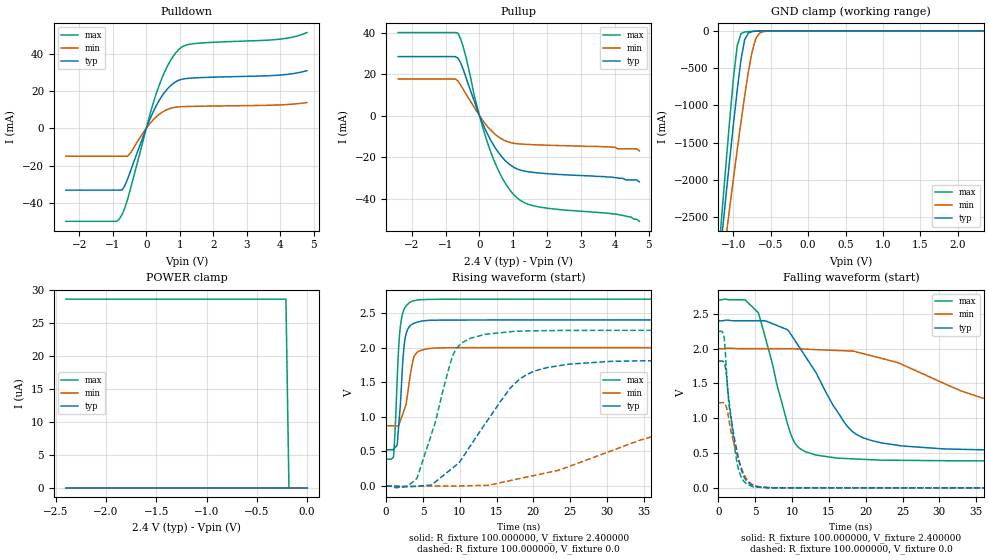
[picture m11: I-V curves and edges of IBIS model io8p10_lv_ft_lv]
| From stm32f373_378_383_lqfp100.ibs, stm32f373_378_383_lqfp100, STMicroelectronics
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|   Model io8p10_lv_ft_lv
[Model]  io8p10_lv_ft_lv
Model_type I/O
Polarity   Non-Inverting
Enable   Active-Low
Vinl =   0.720000V
Vinh =   1.680000V
Vmeas =  1.200000V
Cref =   50.000000pF
Rref =   100.000000M
Vref =   0.0V
C_comp   5.024800pF   4.846300pF   5.260300pF
[Temperature Range]   25.000000   0.125000k   -40.000000
[Pullup Reference]   2.400000V   2.000000V   2.700000V
[Pulldown Reference]   0.0V   0.0V   0.0V
[POWER Clamp Reference]   2.400000V   2.000000V   2.700000V
[GND Clamp Reference]   0.0V   0.0V   0.0V
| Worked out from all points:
|   slope of the pulldown table from 0 to 0.36 V, typ, clamps not added: 25.5 ohm
|   slope of the pullup table from 0 to 0.36 V, typ, clamps not added: 28.4 ohm
|   GND clamp passes 1 mA (typ) near -0.60 V on its own axis
|   rising waveform, R_fixture 100.000000, V_fixture 2.400000: 20-80 % time 716ps typ, 1.14ns min, 631ps max; typ from 0.525 V to 2.4 V
|   rising waveform, R_fixture 100.000000, V_fixture 0.0: 20-80 % time 7.16ns typ, 21ns min, 3.56ns max; typ from 0 V to 1.82 V
|   falling waveform, R_fixture 100.000000, V_fixture 2.400000: 20-80 % time 6.42ns typ, 18.2ns min, 3.43ns max; typ from 2.4 V to 0.525 V
|   falling waveform, R_fixture 100.000000, V_fixture 0.0: 20-80 % time 1.62ns typ, 1.84ns min, 1.36ns max; typ from 1.82 V to 0 V
[Pulldown]
|Voltage   I(typ)   I(min)   I(max)
-2.4V     -33.16mA   -14.98mA   -49.86mA
-880mV    -33.16mA   -14.98mA   -49.86mA
-800mV    -33.16mA   -14.98mA   -48.55mA
-640mV    -30.75mA   -14.98mA   -42.77mA
-480mV    -23.43mA   -13.57mA   -32.92mA
80mV      3.651mA    1.905mA    5.506mA
400mV     15.37mA    7.665mA    23.73mA
720mV     22.75mA    10.69mA    36.23mA
1.04V     26.18mA    11.57mA    43.27mA
1.52V     27.09mA    11.81mA    45.55mA
4V        28.55mA    12.55mA    47.81mA
4.8V      30.9mA     13.81mA    51.31mA
[Pullup]
|Voltage   I(typ)   I(min)   I(max)
-2.4V     28.55mA    17.74mA    40.14mA
-720mV    28.55mA    17.74mA    40.14mA
-640mV    27.85mA    16.83mA    39.87mA
-480mV    22.39mA    12.65mA    33.23mA
-80mV     3.427mA    2.067mA    4.957mA
160mV     -6.219mA   -3.714mA   -9.136mA
320mV     -11.51mA   -6.781mA   -16.98mA
720mV     -21mA      -11.8mA    -31.53mA
1.12V     -25.77mA   -13.54mA   -39.82mA
1.76V     -27.69mA   -14.12mA   -44.06mA
4V        -29.9mA    -15.2mA    -47.5mA
4.72V     -32mA      -17mA      -51mA
[GND_clamp]
|Voltage   I(typ)   I(min)   I(max)
-2.4V     -9.914A    -9.862A    -9.419A
-1.2V     -3.21A     -3.567A    -3.02A
-1.15V    -2.709A    -3.165A    -2.399A
-1.1V     -2.213A    -2.766A    -1.788A
-1.05V    -1.726A    -2.371A    -1.195A
-950mV    -800.5mA   -1.599A    -202.1mA
-900mV    -394.9mA   -1.228A    -38.17mA
-850mV    -120.2mA   -874.5mA   -15.91mA
-750mV    -9.807mA   -279.4mA   -7.273mA
-700mV    -4.736mA   -102mA     -4.51mA
-600mV    -1.032mA   -11.09mA   -922.6uA
2.35V     0A         0A         0A
[POWER_clamp]
|Voltage   I(typ)   I(min)   I(max)
-2.4V     0A         0A         28.66uA
-210mV    0A         0A         28.66uA
-180mV    0A         0A         0A
0V        0A         0A         0A
[Ramp]
| variable   typ   min   max
dV/dt_r  1.09302/7.15321n   0.73320/20.96252n   1.34964/3.55857n
dV/dt_f  1.12473/6.41385n   0.67609/18.23215n   1.38754/3.42182n
R_load = 100.000000
[Rising Waveform]
R_fixture= 100.000000
V_fixture= 2.400000
V_fixture_min= 2.000000
V_fixture_max= 2.700000
|time   V(typ)   V(min)   V(max)
0s        525.2mV    870.3mV    387.4mV
1.001ns   531.4mV    869.3mV    419.4mV
1.301ns   567.1mV    868mV      996.2mV
1.502ns   595.4mV    867.4mV    1.557V
1.902ns   1.139V     935.4mV    2.281V
2.503ns   2.084V     1.116V     2.568V
3.504ns   2.337V     1.735V     2.669V
4.204ns   2.366V     1.932V     2.687V
6.507ns   2.395V     1.992V     2.697V
49.85ns   2.4V       2V         2.7V
[Rising Waveform]
R_fixture= 100.000000
V_fixture= 0.0
V_fixture_min= 0.0
V_fixture_max= 0.0
|time   V(typ)   V(min)   V(max)
0s        4.912nV    72.82nV    3.774nV
4.204ns   -2.416mV   -4.009mV   117.2mV
6.206ns   18.85mV    -735.2uV   767.1mV
9.209ns   277.2mV    -117.8uV   1.92V
13.41ns   892.7mV    10.44mV    2.192V
18.22ns   1.551V     110.3mV    2.237V
24.82ns   1.761V     282.2mV    2.248V
34.63ns   1.809V     667.5mV    2.249V
51.65ns   1.821V     1.101V     2.249V
99.7ns    1.822V     1.223V     2.249V
[Falling Waveform]
R_fixture= 100.000000
V_fixture= 2.400000
V_fixture_min= 2.000000
V_fixture_max= 2.700000
|time   V(typ)   V(min)   V(max)
0s        2.4V       2V         2.7V
3.604ns   2.401V     2.001V     2.702V
5.405ns   2.402V     2V         2.517V
10.01ns   2.178V     2V         721.5mV
13.21ns   1.661V     1.987V     472.4mV
18.22ns   807.9mV    1.965V     417mV
25.03ns   601.2mV    1.769V     395.7mV
35.84ns   547mV      1.291V     387.8mV
47.25ns   530.3mV    1.01V      387.4mV
99.7ns    525.2mV    870.3mV    387.4mV
[Falling Waveform]
R_fixture= 100.000000
V_fixture= 0.0
V_fixture_min= 0.0
V_fixture_max= 0.0
|time   V(typ)   V(min)   V(max)
0s        1.822V     1.223V     2.249V
800.8ps   1.792V     1.218V     2.127V
1.101ns   1.605V     1.153V     1.648V
1.301ns   1.352V     1.054V     1.363V
1.702ns   1V         809.9mV    1.014V
2.503ns   531.1mV    482.6mV    370mV
3.203ns   229.1mV    261.2mV    134.7mV
3.904ns   90.2mV     115.3mV    50.57mV
7.107ns   1.456mV    3.226mV    1.006mV
49.85ns   4.912nV    72.82nV    3.774nV
